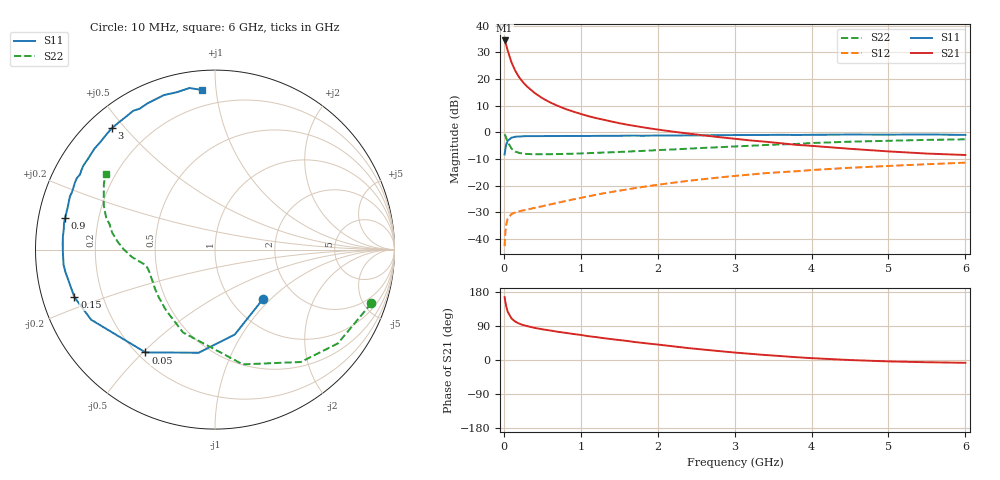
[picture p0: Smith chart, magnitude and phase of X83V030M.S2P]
! SIEMENS Small Signal Semiconductors
! BFP136W
! Si NPN RF Bipolar Junction Transistor in SOT343
! VCE = 3 V  IC = 30 mA
! Common Emitter S-Parameters:  September  1994
# GHz  S  MA  R  50
!  f  S11  S21  S12  S22
! GHz  MAG  ANG  MAG  ANG  MAG  ANG  MAG  ANG
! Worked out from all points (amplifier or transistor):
!   40 points, 10 MHz to 6 GHz, reference 50 ohm
!   highest |S21| = 34.5 dB at 10 MHz (marker M1)
!   |S21| within 3 dB of that: start of sweep to 42.78 MHz
!   unconditionally stable (mu >= 1): 757.4 MHz to 2.818 GHz
!   at 200 MHz: K = 0.43, MSG = 25.1 dB, |S12| = -29.6 dB
!   at 1.5 GHz: K = 1.14, MAG = 10.4 dB, |S12| = -21.9 dB
!   at 6 GHz: K = 0.98, MSG = 1.4 dB, |S12| = -11.4 dB
!   S11 on the Smith chart (normalised r, x): 10 MHz: 1.39, -0.90; 50 MHz: 0.23, -0.51; 150 MHz: 0.10, -0.16; 900 MHz: 0.08, +0.10; 3 GHz: 0.07, +0.46; 6 GHz: 0.10, +0.92
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0.01  0.3838 -45.8  52.88 165.9  0.0073 74.8  0.9213 -18.9
0.02  0.4859 -76.9  48.31 153.0  0.0134 64.5  0.8614 -37.3
0.03  0.5819 -99.0  43.84 142.6  0.0185 56.2  0.7882 -52.6
0.05  0.6916 -124.1  34.24 127.4  0.0239 42.1  0.6578 -76.4
0.1  0.7931 -150.5  20.4 109.4  0.0294 30.9  0.4949 -111.1
0.15  0.8271 -161.3  14.14 101.0  0.0313 28.7  0.4343 -129.0
0.2  0.8326 -167.2  10.71 95.9  0.033 28.1  0.4106 -139.7
0.25  0.8429 -171.6  8.671 92.3  0.0342 29.2  0.3993 -146.7
0.3  0.8481 -174.3  7.263 89.6  0.0353 30.7  0.3919 -151.4
0.4  0.8477 -179.1  5.479 84.8  0.0382 33.9  0.3874 -157.5
0.5  0.8491 177.7  4.369 81.0  0.041 37.5  0.3868 -161.4
0.6  0.8505 175.1  3.647 77.9  0.0442 39.9  0.3881 -163.6
0.7  0.8502 172.2  3.138 74.5  0.0476 43.3  0.3905 -165.1
0.9  0.8534 168.2  2.455 68.7  0.055 47.2  0.3967 -167.5
1.1  0.8541 163.6  2.005 62.8  0.063 50.0  0.4063 -168.8
1.6  0.865 154.5  1.392 50.4  0.0845 53.4  0.4345 -172.0
2.2  0.8699 144.2  1.028 36.1  0.1131 52.9  0.4763 -176.4
3  0.8876 130.3  0.757 19.7  0.1517 48.1  0.5426 175.6
3.2  0.8888 126.8  0.705 16.4  0.1609 46.5  0.5585 173.3
4.5  0.9067 108.3  0.49 -0.1  0.2159 35.1  0.6665 158.4
5.5  0.9114 99.0  0.399 -5.9  0.2518 27.1  0.72 149.3
6  0.8924 94.6  0.375 -7.4  0.2692 22.6  0.7389 145.4
